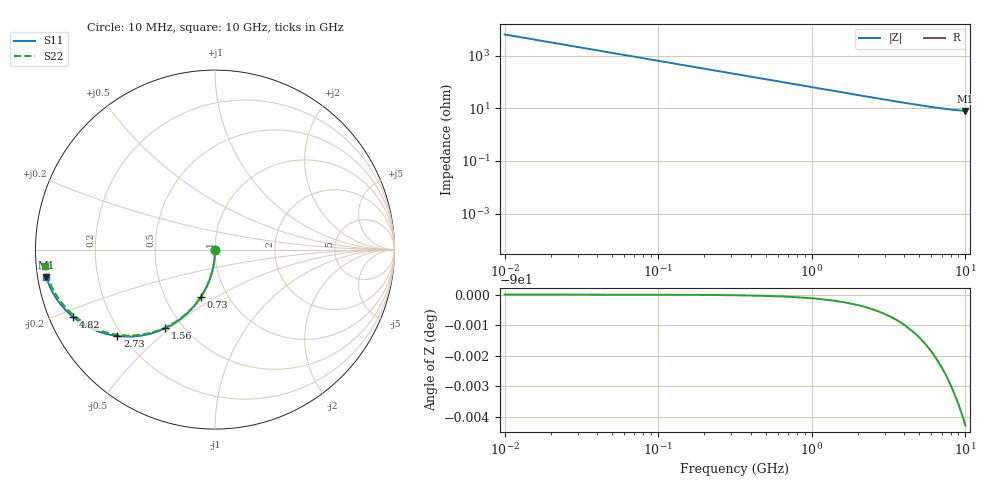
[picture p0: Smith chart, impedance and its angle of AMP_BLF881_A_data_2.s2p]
! Created Tue Feb 16 10:30:37 2010
# ghz S ma R 50
! 2 Port Network Data from SP1.SP block
! freq  magS11  angS11  magS21  angS21  magS12  angS12  magS22  angS22
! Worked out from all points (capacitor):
!   1000 points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, 10 MHz to 10 GHz, reference 50 ohm
!   read as one part in shunt: C = 2.53 pF near 60 MHz
!   lowest |Z| = 7.87 ohm at 10 GHz (marker M1)
!   S11 on the Smith chart (normalised r, x): 10 MHz: 1.00, -0.01; 730 MHz: 0.75, -0.43; 1.56 GHz: 0.40, -0.48; 2.73 GHz: 0.18, -0.37; 4.82 GHz: 0.07, -0.22; 10 GHz: 0.02, -0.08
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0.01  0.003906 -90.2  1 -0.2  1 -0.2  0.003906 -90.2
0.04  0.01562 -90.9  0.9999 -0.9  0.9999 -0.9  0.01562 -90.9
0.07  0.02733 -91.6  0.9996 -1.6  0.9996 -1.6  0.02733 -91.6
0.09  0.03513 -92.1  0.9994 -2.1  0.9994 -2.1  0.03513 -92.1
0.11  0.04293 -92.5  0.9991 -2.6  0.9991 -2.6  0.04293 -92.6
0.14  0.05461 -93.2  0.9985 -3.2  0.9985 -3.2  0.05461 -93.3
0.2  0.07789 -94.6  0.997 -4.6  0.997 -4.6  0.07789 -94.7
0.29  0.1126 -96.7  0.9936 -6.7  0.9936 -6.7  0.1126 -96.7
0.41  0.1582 -99.4  0.9874 -9.4  0.9874 -9.4  0.1582 -99.5
0.56  0.2137 -102.7  0.9769 -12.8  0.9769 -12.8  0.2137 -102.9
0.73  0.2742 -106.4  0.9617 -16.5  0.9617 -16.5  0.2742 -106.6
1.1  0.3946 -114.0  0.9188 -24.2  0.9188 -24.2  0.3946 -114.3
1.56  0.5197 -122.4  0.8543 -32.6  0.8543 -32.6  0.5197 -122.9
1.68  0.5478 -124.4  0.8366 -34.6  0.8366 -34.6  0.5478 -124.9
2.16  0.643 -131.5  0.7659 -41.9  0.7659 -41.9  0.643 -132.2
2.73  0.7262 -138.5  0.6875 -48.9  0.6875 -48.9  0.7262 -139.3
3.34  0.7888 -144.4  0.6146 -55.0  0.6146 -55.0  0.7888 -145.5
4.82  0.875 -154.6  0.4841 -65.3  0.4841 -65.3  0.875 -156.1
5.01  0.8819 -155.5  0.4714 -66.4  0.4714 -66.4  0.8819 -157.2
6.67  0.9221 -162.3  0.3868 -73.4  0.3868 -73.4  0.9221 -164.6
8.34  0.9419 -167.1  0.3357 -78.5  0.3357 -78.5  0.9419 -170.0
10  0.952 -170.7  0.3059 -82.5  0.3059 -82.5  0.952 -174.3
